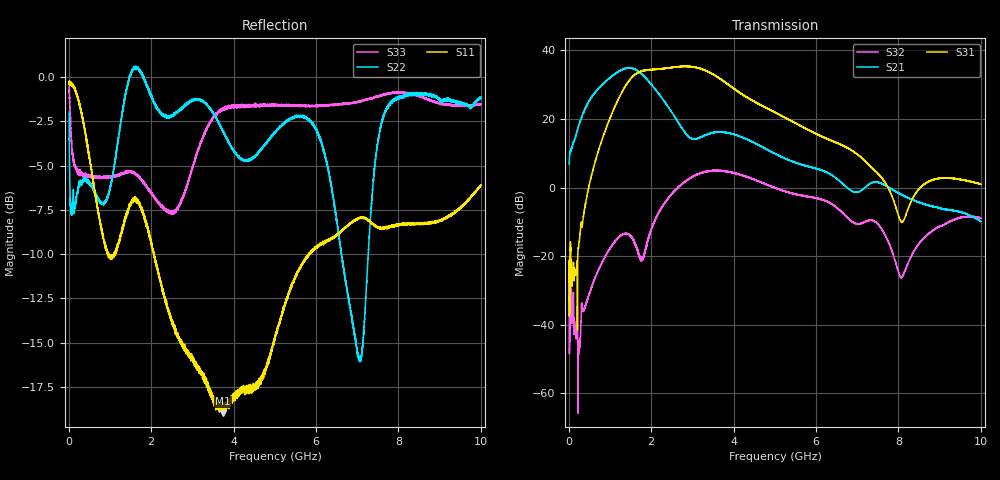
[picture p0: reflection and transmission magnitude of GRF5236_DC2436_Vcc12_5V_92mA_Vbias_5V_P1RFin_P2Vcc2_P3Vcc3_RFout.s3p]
!Keysight Technologies,N5245B,MY56052315,A.20.20.05
!Date: Friday, August 21, 2026 13:49:22
!Correction: S11(C  3-Port  )
!S12(C  3-Port  )
!S13(C  3-Port  )
!S21(C  3-Port  )
!S22(C  3-Port  )
!S23(C  3-Port  )
!S31(C  3-Port  )
!S32(C  3-Port  )
!S33(C  3-Port  )
!S3P File: Measurements: <S11,S12,S13>,
!<S21,S22,S23>,
!<S31,S32,S33>:
# Hz S  RI  R 50
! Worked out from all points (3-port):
!   9991 points, 10 MHz to 10 GHz, reference 50 ohm
!   strongest paths, dB at 10 MHz, 2.507 GHz, 5.005 GHz, 7.503 GHz, 10 GHz:
!     S31: -27.7, 35.0, 21.9, 4.0, 1.0
!     S21: 6.8, 21.8, 9.9, 1.5, -9.9
!     S32: -35.2, -1.8, 0.0, -10.7, -9.0
!   lowest |S11| = -19.0 dB at 3.744 GHz (marker M1), VSWR 1.25, Z = 51.6 + j11.4 ohm
!   |S11| at or under -10 dB: 970.1 MHz to 1.092 GHz (121.5 MHz wide, 11.8 % of centre); 2.065119 GHz to 2.071704 GHz (6.585 MHz wide, 0.318 % of centre); 2.072 GHz to 5.821 GHz (3.748 GHz wide, 95 % of centre)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
1e7  0.9564 -0.0297  0.000336 0.000172  -0.00153 -0.000383
     0.8416 2.021  0.4385 -0.6638  -0.000758 -0.0011
     -0.0108 -0.0396  0.0156 0.00775  0.8987 -0.3534
6.65e8  -0.0244 -0.4471  -0.00164 0.00874  -0.000297 0.00053
        22.86 11.06  -0.4551 0.099  0.00431 -0.00836
        2.64 0.3195  0.0526 0.00432  -0.5173 -0.0554
1.16e9  -0.0946 -0.3074  0.000597 0.0125  -0.000111 0.0011
        40.92 -23.26  -0.5871 -0.1892  -0.0203 -0.0245
        10.94 -12.95  0.0848 -0.1502  -0.5254 -0.0141
1.527e9  -0.3579 -0.2602  0.000215 0.0172  -5.05e-05 0.00166
         2.222 -54.95  -1.031 -0.0362  -0.051 0.0107
         -15.32 -37.03  -0.1393 -0.1289  -0.5374 0.0249
1.977e9  -0.2986 0.1812  0.00499 0.0206  0.000463 0.00132
         -30.23 -14.2  -0.7556 0.4839  -0.00657 0.0382
         -51.62 6.649  0.2114 0.0531  -0.4707 0.0555
2.777e9  0.023 0.17  0.0041 0.0218  0.000775 0.00169
         -6.593 2.01  -0.6111 0.5522  -0.00335 0.0155
         7.654 58.22  -0.1534 -1.15  -0.4476 -0.1059
3.249e9  0.0656 0.1271  0.00169 0.026  0.000608 0.00185
         -5.481 -0.8843  -0.6094 0.5978  -0.00501 0.0293
         47.03 24.5  -1.446 -0.7921  -0.6594 -0.1338
3.744e9  0.0281 0.1086  0.0009 0.0334  0.000554 0.00193
         -6.317 0.9813  -0.4494 0.5359  0.0141 0.0351
         33.01 -14.64  -1.592 0.6649  -0.8069 0.072
5.005e9  -0.1468 0.1074  0.011 0.0415  0.00101 0.00243
         -1.518 2.729  -0.2685 0.6446  0.0261 0.00813
         -1.952 -12.33  0.303 0.9486  -0.7818 0.2856
1e10  -0.0877 0.4876  0.0339 0.0328  0.000588 0.000434
      0.2178 0.2344  -0.104 0.8691  0.0237 0.00323
      -0.9682 0.5602  0.3501 -0.0585  0.2984 0.7857
